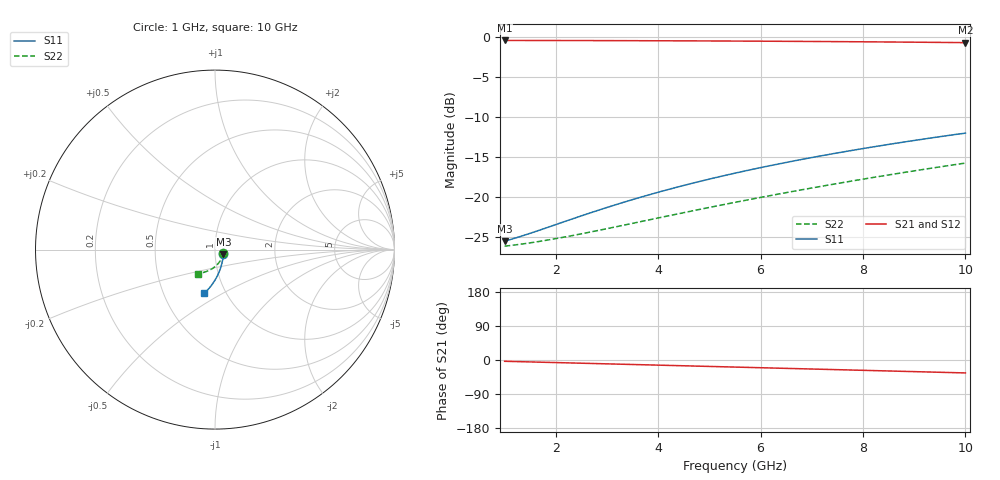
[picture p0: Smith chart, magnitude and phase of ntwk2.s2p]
! Created Thu Nov 11 11:10:01 2010
# ghz S ri R 50
! 2 Port Network Data from SP1.SP block
! freq  reS11  imS11  reS21  imS21  reS12  imS12  reS22  imS22
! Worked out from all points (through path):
!   91 points, 1 GHz to 10 GHz, reference 50 ohm
!   highest |S21| = -0.43 dB at 1 GHz (marker M1); lowest = -0.7 dB at 10 GHz (marker M2)
!   group delay of S21, straight-line fit = 9.49 ps
!   lowest |S11| = -25.5 dB at 1 GHz (marker M3), VSWR 1.11, Z = 54.8 - j2.86 ohm
!   |S11| at or under -10 dB: start of sweep to end of sweep
!   |S22| runs from -26.1 to -15.7 dB; largest |S21 - S12| = 0
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1  0.0466 -0.026  0.9504 -0.0562  0.9504 -0.0562  0.0461 -0.0185
1.3  0.0459 -0.0338  0.9491 -0.0731  0.9491 -0.0731  0.045 -0.024
1.5  0.0453 -0.039  0.948 -0.0843  0.948 -0.0843  0.0442 -0.0276
1.7  0.0446 -0.0441  0.9468 -0.0955  0.9468 -0.0955  0.0432 -0.0312
2.1  0.043 -0.0545  0.9438 -0.1178  0.9438 -0.1178  0.0408 -0.0384
2.5  0.0411 -0.0648  0.9403 -0.14  0.9403 -0.14  0.038 -0.0455
2.9  0.0388 -0.0751  0.9361 -0.1621  0.9361 -0.1621  0.0347 -0.0524
3.3  0.0362 -0.0853  0.9313 -0.1841  0.9313 -0.1841  0.031 -0.0592
3.6  0.034 -0.093  0.9273 -0.2005  0.9273 -0.2005  0.0278 -0.0642
4  0.0308 -0.1032  0.9215 -0.2223  0.9215 -0.2223  0.0232 -0.0707
4.3  0.0282 -0.1108  0.9167 -0.2385  0.9167 -0.2385  0.0195 -0.0754
4.7  0.0243 -0.1208  0.9098 -0.2599  0.9098 -0.2599  0.0141 -0.0816
5.1  0.0202 -0.1308  0.9023 -0.2812  0.9023 -0.2812  0.00826 -0.0875
5.5  0.0156 -0.1408  0.8942 -0.3022  0.8942 -0.3022  0.00199 -0.0931
5.8  0.012 -0.1481  0.8877 -0.3178  0.8877 -0.3178  -0.00299 -0.0972
6.2  0.00685 -0.1579  0.8786 -0.3384  0.8786 -0.3384  -0.01 -0.1023
6.6  0.00134 -0.1676  0.8689 -0.3587  0.8689 -0.3587  -0.0174 -0.1071
7  -0.00454 -0.1772  0.8586 -0.3787  0.8586 -0.3787  -0.0252 -0.1116
7.7  -0.0157 -0.1936  0.8392 -0.413  0.8392 -0.413  -0.0398 -0.1187
8.5  -0.0298 -0.2119  0.815 -0.4509  0.815 -0.4509  -0.0579 -0.1253
9.2  -0.0434 -0.2273  0.792 -0.4828  0.792 -0.4828  -0.0747 -0.1298
10  -0.0604 -0.2443  0.7638 -0.5178  0.7638 -0.5178  -0.0951 -0.1332
